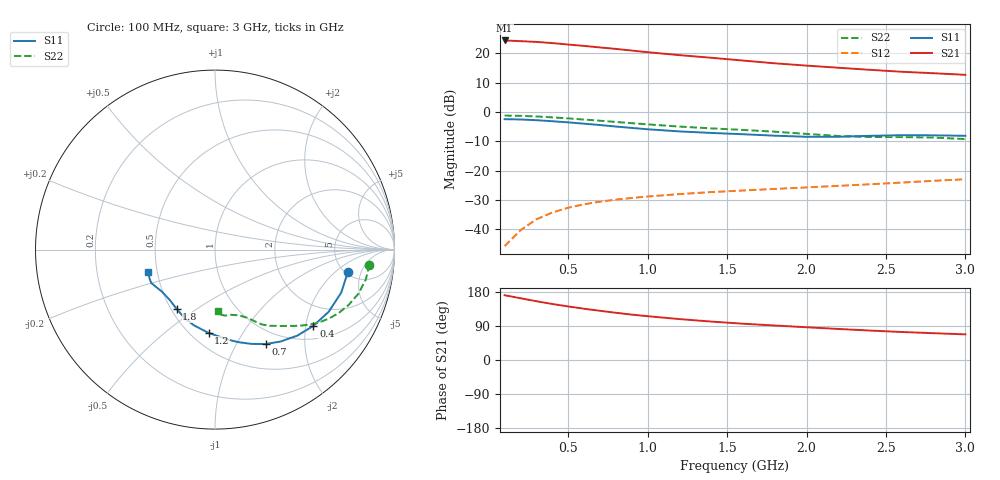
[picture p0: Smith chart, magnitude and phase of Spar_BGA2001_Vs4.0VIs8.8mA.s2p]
! Filename: 4G1.00101
! Title: BGA2001 X0297-20 HFE=80
! Bias: Vce=4.0V,Ic=8.8mA
! Company: NXP Semiconductors NL
! User: Quality&Reliability T&D
! Measure time: 23 Oct 1998 / 09:21:29
#  MHz  S  MA  R 50
! Freq  S11  S21  S12  S22  :
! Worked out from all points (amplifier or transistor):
!   20 points, 100 MHz to 3 GHz, reference 50 ohm
!   highest |S21| = 24.3 dB at 100 MHz (marker M1)
!   |S21| within 3 dB of that: start of sweep to 821.4 MHz
!   unconditionally stable (mu >= 1): 1.763 GHz to end of sweep
!   at 400 MHz: K = 0.37, MSG = 28.9 dB, |S12| = -34.3 dB
!   at 1.2 GHz: K = 0.75, MSG = 23.7 dB, |S12| = -28.0 dB
!   at 3 GHz: K = 1.25, MAG = 14.8 dB, |S12| = -22.9 dB
!   S11 on the Smith chart (normalised r, x): 100 MHz: 5.31, -2.98; 400 MHz: 1.35, -2.21; 700 MHz: 0.81, -1.33; 1.2 GHz: 0.61, -0.72; 1.8 GHz: 0.53, -0.42; 3 GHz: 0.45, -0.13
100  0.751 -9.4  16.46 170.9  0.005168 67.5  0.8644 -5.5
200  0.743 -18.8  16.02 163.0  0.009652 75.0  0.8566 -11.2
300  0.7223 -28.5  15.55 155.1  0.0148 74.3  0.8357 -17.1
400  0.6936 -37.8  14.85 147.8  0.01932 71.0  0.8062 -22.4
500  0.6632 -46.3  14.03 141.3  0.02332 67.7  0.7743 -27.2
600  0.6297 -54.4  13.29 135.3  0.02669 65.0  0.7405 -31.4
700  0.5975 -61.7  12.51 129.8  0.02961 62.7  0.7075 -35.0
800  0.5634 -68.9  11.82 124.6  0.03208 60.8  0.6747 -38.2
900  0.5331 -75.5  11.08 119.8  0.03416 59.4  0.6429 -41.1
1000  0.5061 -82.0  10.39 115.6  0.03624 58.5  0.6131 -43.9
1200  0.4653 -94.4  9.257 108.0  0.0398 57.2  0.5618 -49.2
1400  0.4382 -105.5  8.357 101.4  0.04308 56.7  0.5245 -54.1
1600  0.4164 -114.3  7.483 95.7  0.04587 57.3  0.493 -57.9
1800  0.3934 -122.9  6.719 91.1  0.04878 58.7  0.4596 -60.8
2000  0.3769 -132.4  6.138 86.3  0.05177 59.3  0.4215 -64.5
2200  0.3774 -141.8  5.646 81.9  0.05498 59.6  0.3894 -70.0
2400  0.3909 -148.5  5.205 77.7  0.05852 60.5  0.3736 -76.5
2600  0.4011 -152.5  4.823 73.9  0.0626 62.0  0.3719 -81.4
2800  0.3985 -156.3  4.553 70.7  0.06706 62.3  0.3654 -84.3
3000  0.3918 -161.5  4.276 67.6  0.07128 62.9  0.3444 -87.1
